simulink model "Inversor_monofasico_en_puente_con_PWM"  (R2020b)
settings: Solver=FixedStepAuto  StartTime=0.0  StopTime=0.06  FixedStep=0.00001  RelTol=1e-3
undefined symbols (not defined in the file): Bipolar, bridge, full, modulation, phase, pulses, Single
libraries: powerlib x14, powerlib_meascontrol x3, simulink x1

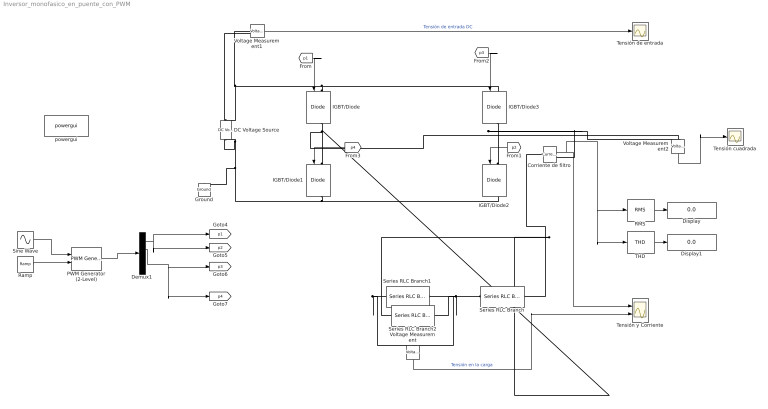
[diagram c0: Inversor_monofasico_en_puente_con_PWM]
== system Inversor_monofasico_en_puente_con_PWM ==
  Corriente de filtro : powerlib/Measurements/Current Measurement  PhasorSimulation=off  OutputType=Complex  PSBequivalent=0
  DC Voltage Source : powerlib/Electrical Sources/DC Voltage Source  Amplitude=36  Measurements=Voltage
  Demux1 : Demux
  Display : Display
  Display1 : Display
  Ground : powerlib/Elements/Ground  LConnTagsString=a
  IGBT/Diode{,1..3} (4 alike) : powerlib/Power Electronics/IGBT//Diode  Ron=1e-3  Rs=1e5  Cs=inf  Measurements=on
  PWM Generator (2-Level) : powerlib_meascontrol/Pulse & Signal Generators/PWM Generator (2-Level)  ModulatorType=Single-phase full-bridge - Bipolar modulation (4 pulses)  ModulatorMode=Synchronized  Fc=27*60  Pc=90  nF=39  MinMax="[ -1.2  1.2 ]"  SamplingTechnique=Natural  ModulatingSignals=off  m=0.8  Freq=60  Phase=0  Ts=0  ShowCarrierOutport=off
  RMS : powerlib_meascontrol/Measurements/RMS  TrueRMS=on  Freq=50  RMSInit=120  Ts=0
  Ramp : simulink/Sources/Ramp  slope=2*pi*50  start=0  InitialOutput=0
  Series RLC Branch : powerlib/Elements/Series RLC Branch  LConnTagsString=__new0  RConnTagsString=__new0  BranchType=RL  Resistance=0.001  Inductance=0.010  SetiL0=off  InitialCurrent=0  Capacitance=1e-6  Setx0=off  InitialVoltage=0  Measurements=None
  Series RLC Branch1 : powerlib/Elements/Series RLC Branch  LConnTagsString=__new0  RConnTagsString=__new0  BranchType=C  Resistance=10  Inductance=0.005  SetiL0=off  InitialCurrent=0  Capacitance=1e-3  Setx0=off  InitialVoltage=0  Measurements=None
  Series RLC Branch2 : powerlib/Elements/Series RLC Branch  LConnTagsString=__new0  RConnTagsString=__new0  BranchType=RL  Resistance=4  Inductance=0.001  SetiL0=off  InitialCurrent=0  Capacitance=1e-6  Setx0=off  InitialVoltage=0  Measurements=None
  Sine Wave : Sin  Frequency=2*pi*50  SampleTime=0
  THD : powerlib_meascontrol/Measurements/THD  Freq=50  Ts=0
  Tensión cuadrada : Scope
  Tensión de entrada : Scope
  "Tensión y Corriente " : Scope  NumInputPorts=2
  Voltage Measurement : powerlib/Measurements/Voltage Measurement  PhasorSimulation=off  OutputType=Complex  PSBequivalent=0
  Voltage Measurement1 : powerlib/Measurements/Voltage Measurement  PhasorSimulation=off  OutputType=Complex  PSBequivalent=0
  Voltage Measurement2 : powerlib/Measurements/Voltage Measurement  PhasorSimulation=off  OutputType=Complex  PSBequivalent=0
  powergui : powerlib/powergui  Priority=1  SimulationMode=Continuous  SampleTime=50e-6  frequency=60  Iterations=50  frequencyindice=0  Pbase=100e6  ErrMax=1e-4  UnitsV=kV  UnitsW=MW  buscounter=0  FunctionMessages=off  echomessages=off  EnableUseOfTLC=off  CurrentSourceSwitches=off  DisableSnubberDevices=off  DisableRonSwitches=off  DisableVfSwitches=off  DisplayEquations=off  AutomaticDiscreteSolvers=off  SolverType=Tustin/Backward Euler (TBE)  Interpol=off  ExternalGateDelay=off  methode=off  Ts=100  x0status=blocks  SPID=on  SwTol=0  HookPort=off  NonlinearTolerance=1e-4  nMaxIteration=100  ContinueOnMaxIteration=off  RestoreLinks=warning  ResistiveCurrentMeasurement=off  Frange=[0:2:500]  Ylog=off  Xlog=on  ShowGrid=off  save=off  variable=ZData  structure=0  ZoomFFT=off  StartTime=0.0  cycles=1  DisplayStyle=1  fundamental=60  FreqAxis=off  MaxFrequency=1000  frequencyindicesteady=1  RmsSteady=1  display=off
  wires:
  [p1] -> IGBT/Diode/1
  [p3] -> IGBT/Diode3/1
  [p2] -> IGBT/Diode2/1
  [p4] -> IGBT/Diode1/1
  Sine Wave/1 -> PWM Generator (2-Level)/1
  Demux1/1 -> [p2], [p1]
  PWM Generator (2-Level)/1 -> Demux1/1
  Demux1/2 -> [p3], [p4]
  Corriente de filtro/1 -> THD/1, RMS/1, "Tensión y Corriente "/1
  Ramp/1 -> PWM Generator (2-Level)/2
  RMS/1 -> Display/1
  THD/1 -> Display1/1
  Voltage Measurement1/1 -> Tensión de entrada/1  "Tensión de entrada DC"
  Voltage Measurement/1 -> "Tensión y Corriente "/2  "Tensión en la carga"
  Voltage Measurement2/1 -> Tensión cuadrada/1
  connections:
  IGBT/Diode/RConn1 -- Series RLC Branch2/LConn1 -- Voltage Measurement/LConn2 -- Series RLC Branch1/LConn1 -- Voltage Measurement2/LConn1 -- IGBT/Diode1/LConn1
  Corriente de filtro/LConn1 -- Series RLC Branch/RConn1
  IGBT/Diode/LConn1 -- IGBT/Diode3/LConn1 -- DC Voltage Source/RConn1 -- Voltage Measurement1/LConn1
  IGBT/Diode1/RConn1 -- IGBT/Diode2/RConn1 -- Ground/LConn1 -- Voltage Measurement1/LConn2 -- DC Voltage Source/LConn1
  IGBT/Diode3/RConn1 -- Voltage Measurement2/LConn2 -- Corriente de filtro/RConn1 -- IGBT/Diode2/LConn1
  Series RLC Branch1/RConn1 -- Series RLC Branch2/RConn1 -- Voltage Measurement/LConn1 -- Series RLC Branch/LConn1
